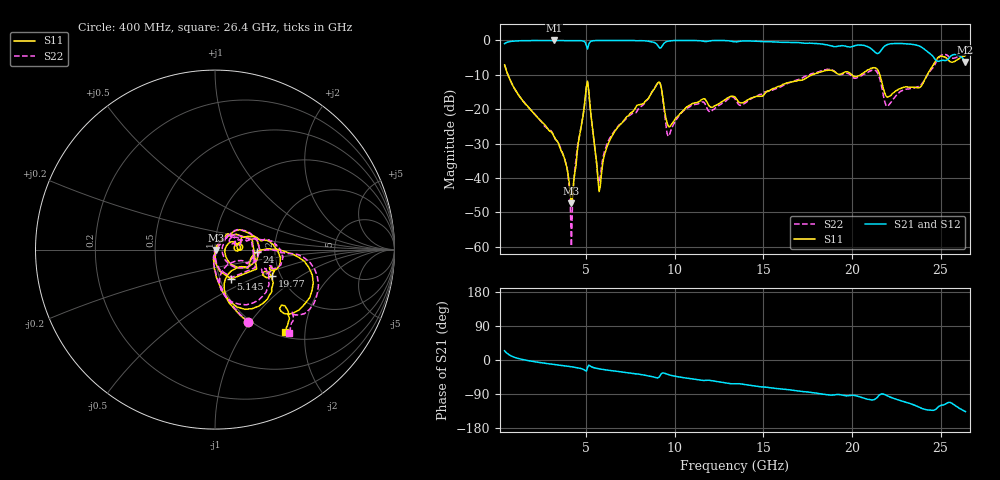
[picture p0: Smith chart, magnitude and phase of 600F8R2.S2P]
!  American Technical Ceramics  Date:  11/23/05
!  One Norden Lane
!  Huntington Station,  NY.  11746-2102
!  Tel:  (631) 622-4700  Fax:  (631) 622-4748
!  Part Number  600F8R2  Mounting Orientation: Horizontal
!  Description: Ultra Low ESR Microwave capacitors
!  Application: Coupling, Bypass, Tuning, DC Block
!  Filters, Matching
# GHZ S DB R 50
! Freq  |S11|  S11 Ph  |S21|  S21 Ph  |S12|  S12 Ph  |S22|  S22 Ph
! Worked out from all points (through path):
!   401 points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, 400 MHz to 26.4 GHz, reference 50 ohm
!   highest |S21| = 0.00 dB at 3.195 GHz (marker M1); lowest = -6.2 dB at 26.4 GHz (marker M2)
!   group delay of S21, straight-line fit = 14.3 ps
!   lowest |S11| = -47.4 dB at 4.17 GHz (marker M3), VSWR 1.01, Z = 50.4 - j0.184 ohm
!   |S11| at or under -10 dB: 587 MHz to 17.76 GHz (17.17 GHz wide, 187 % of centre); 20 GHz to 20.48 GHz (483.5 MHz wide, 2.39 % of centre); 21.57 GHz to 24.25 GHz (2.679 GHz wide, 11.7 % of centre)
!   |S22| runs from -59.9 to -4.0 dB; largest |S21 - S12| = 0.0088
!   S11 on the Smith chart (normalised r, x): 400 MHz: 0.97, -0.97; 5.145 GHz: 1.13, -0.38; 19.77 GHz: 1.81, -0.60; 24 GHz: 1.61, -0.04; 26.4 GHz: 1.10, -1.58
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0.4  -7.10 -65.6  -0.93 24.4  -0.94 24.3  -7.10 -65.2
3.195  -27.99 -97.6  0.00 -11.8  0.00 -11.8  -27.97 -101.9
3.845  -35.58 -87.6  -0.01 -15.8  -0.01 -15.8  -35.54 -101.0
4.17  -47.42 -25.4  -0.02 -17.9  -0.03 -17.9  -59.85 158.8
4.755  -24.24 53.2  -0.09 -23.1  -0.10 -23.2  -24.09 55.1
5.015  -13.37 14.9  -1.48 -29.3  -1.49 -29.1  -13.53 15.3
5.145  -14.58 -61.3  -1.18 -13.3  -1.19 -13.7  -14.83 -58.9
5.6  -35.95 -79.2  -0.01 -22.1  -0.01 -22.1  -36.25 -70.3
5.795  -42.54 16.8  -0.01 -23.9  -0.01 -23.9  -39.70 14.1
6.51  -27.37 53.7  -0.01 -28.5  -0.01 -28.6  -26.97 46.5
9.11  -12.07 -0.4  -1.96 -45.4  -1.93 -45.3  -12.06 -0.6
9.695  -25.18 -4.1  -0.14 -39.4  -0.15 -39.3  -27.56 14.9
10.865  -18.76 21.3  0.00 -49.0  0.00 -49.1  -19.23 42.1
13.4  -16.47 0.8  -0.37 -62.7  -0.38 -62.8  -16.99 11.5
17.755  -10.01 6.5  -0.84 -86.1  -0.86 -86.1  -9.64 6.7
19.77  -9.12 -24.4  -1.82 -94.5  -1.84 -94.6  -9.61 -21.9
21.33  -8.01 -52.5  -3.56 -102.5  -3.55 -102.5  -8.75 -54.5
22.11  -16.20 -44.0  -1.05 -96.8  -1.07 -96.9  -18.58 -37.9
23.995  -12.57 -2.9  -2.21 -128.7  -2.21 -128.6  -12.34 -4.0
25.035  -4.56 -26.8  -5.81 -119.6  -5.81 -119.7  -4.31 -18.8
25.75  -6.18 -39.4  -4.09 -117.9  -4.12 -117.9  -5.16 -39.1
26.4  -4.40 -49.5  -6.22 -136.1  -6.24 -136.1  -4.15 -48.4
